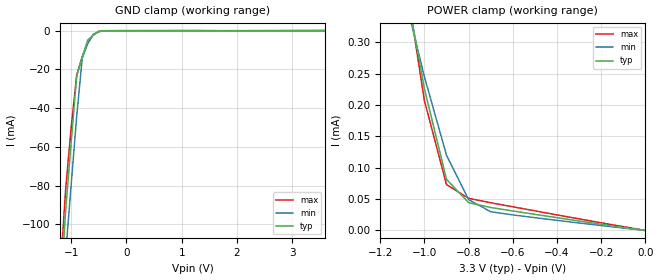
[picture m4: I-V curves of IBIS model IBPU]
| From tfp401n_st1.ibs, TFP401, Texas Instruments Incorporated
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|   INPUT  MODEL WITH PULL UP
[Model]   IBPU
Model_type   Input
| Signals   PDOZ, PDZ, RSVD
Vinl = 1.08
Vinh = 2.10
| variable   typ   min   max
C_comp   2pF   NA   NA
|   typ   min   max
[Temperature Range] 25.0   70.0   0.0
[Voltage range]   3.3V   3.0V   3.6V
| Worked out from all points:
|   GND clamp passes 1 mA (typ) near -0.54 V on its own axis
|   POWER clamp passes 1 mA (typ) near -1.36 V on its own axis
[GND_clamp]
|Voltage   I(typ)   I(min)   I(max)
-3.6V     -1.31A     -1.33A     -1.29A
-1.2V     -138mA     -161mA     -126mA
-1.1V     -92.5mA    -115mA     -81.5mA
-1V       -57.2mA    -79.3mA    -49.9mA
-900mV    -23.2mA    -44mA      -22.8mA
-800mV    -13.6mA    -14.2mA    -13.5mA
-700mV    -4.81mA    -6.63mA    -6.24mA
-600mV    -2.31mA    -1.89mA    -2.24mA
-500mV    -238uA     -530uA     -465uA
-300mV    -47.3uA    -35.1uA    -67.2uA
3.6V      15.1uA     24.8uA     1.33nA
[Power_clamp]
|Note that the [Power_clamp] voltage table is referenced to Vcc
|and is calculated using Vtable=Vcc-Vmeasured.
|Voltage   I(typ)   I(min)   I(max)
-3.3V     5.6mA      4.03mA     6.88mA
-1.1V     419uA      389uA      435uA
-1V       226uA      245uA      207uA
-900mV    81.5uA     120uA      73.1uA
-800mV    44.3uA     49.2uA     51.2uA
-700mV    36.6uA     29.8uA     44.2uA
0V        35.3pA     99.7pA     34.3pA
